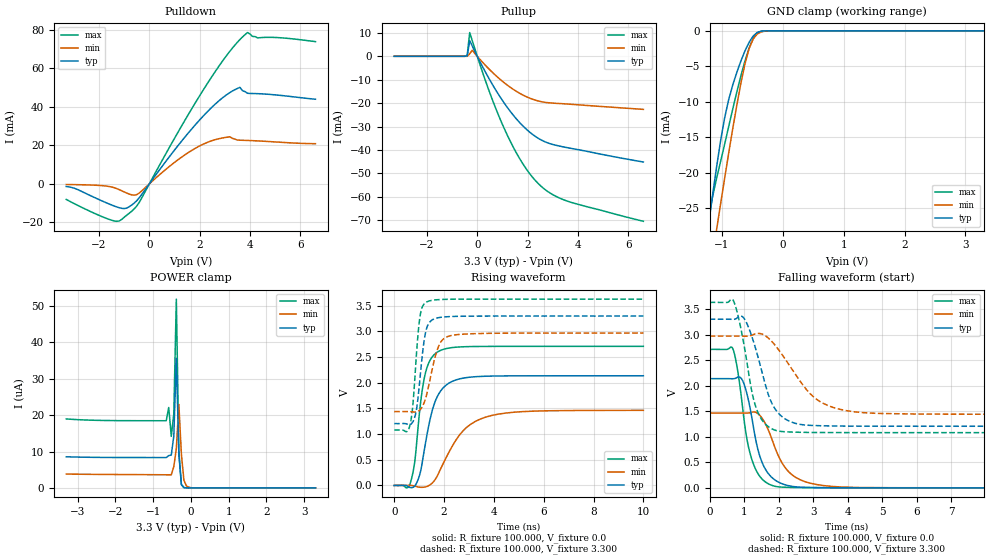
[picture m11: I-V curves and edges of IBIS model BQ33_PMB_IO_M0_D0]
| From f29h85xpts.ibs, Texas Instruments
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|   Model BQ33_PMB_IO_M0_D0
[Model]   BQ33_PMB_IO_M0_D0
Model_type   I/O
Polarity   Non-Inverting
Enable   Active-Low
Vinl =   0.990V
Vinh =   2.310V
Vmeas =  1.650V
Cref =   10.000pF
Vref =   0.0V
|   typ   min   max
C_comp   1.786pF   1.720pF   1.856pF
[Model Spec]
Vinh   2.310V   2.079V   2.541V
Vinl   0.990V   0.891V   1.089V
[Temperature Range]   30   155   -40
[Voltage Range]   3.300V   2.970V   3.630V
[Pullup Reference]   3.300V   2.970V   3.630V
[Pulldown Reference]   0.0V   0.0V   0.0V
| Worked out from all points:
|   slope of the pulldown table from 0 to 0.495 V, typ, clamps not added: 55.8 ohm
|   slope of the pullup table from 0 to 0.495 V, typ, clamps not added: 49.3 ohm
|   GND clamp passes 1 mA (typ) near -0.51 V on its own axis
|   rising waveform, R_fixture 100.000, V_fixture 0.0: 20-80 % time 590ps typ, 1.18ns min, 399ps max; typ from 0 V to 2.14 V
|   rising waveform, R_fixture 100.000, V_fixture 3.300: 20-80 % time 286ps typ, 457ps min, 238ps max; typ from 1.21 V to 3.3 V
|   falling waveform, R_fixture 100.000, V_fixture 0.0: 20-80 % time 441ps typ, 650ps min, 388ps max; typ from 2.14 V to 0 V
|   falling waveform, R_fixture 100.000, V_fixture 3.300: 20-80 % time 565ps typ, 1.03ns min, 431ps max; typ from 3.3 V to 1.21 V
[Pulldown]
|Voltage   I(typ)   I(min)   I(max)
-3.3V     -1.377mA   -342.6uA   -8.105mA
-1.6V     -10.44mA   -1.363mA   -18.44mA
-1.1V     -12.71mA   -3.581mA   -18.49mA
-500mV    -8.748mA   -5.592mA   -11.5mA
1.3V      22.5mA     14.05mA    30.49mA
2.5V      39.99mA    22.49mA    56.04mA
3.2V      47.44mA    24.45mA    68.91mA
3.5V      49.58mA    22.74mA    73.6mA
3.8V      47.94mA    22.6mA     77.52mA
3.9V      47.06mA    22.56mA    78.61mA
4.3V      46.87mA    22.32mA    75.86mA
6.6V      43.98mA    20.88mA    73.9mA
[Pullup]
|Voltage   I(typ)   I(min)   I(max)
-3.3V     194.8pA    13.15nA    1.362nA
-500mV    17.31nA    18.01nA    59.06nA
-400mV    178uA      374.8nA    408.1uA
-300mV    6.695mA    1.073mA    10.14mA
-200mV    4.421mA    2.585mA    6.742mA
400mV     -8.225mA   -4.706mA   -12.71mA
1V        -18.86mA   -10.69mA   -29.11mA
1.7V      -28.49mA   -15.89mA   -44mA
2.3V      -34.18mA   -18.71mA   -52.97mA
2.8V      -37mA      -19.82mA   -57.77mA
3.5V      -38.88mA   -20.34mA   -61.58mA
6.6V      -45.18mA   -22.68mA   -70.51mA
[GND_clamp]
|Voltage   I(typ)   I(min)   I(max)
-3.3V     -172.4mA   -157.9mA   -199.3mA
-1.223V   -27.66mA   -35.7mA    -26.88mA
-1.156V   -23.42mA   -31.92mA   -23.54mA
-1.089V   -19.35mA   -28.18mA   -20.9mA
-1.022V   -15.58mA   -24.48mA   -18.47mA
-955mV    -12.3mA    -20.84mA   -16.02mA
-821mV    -7.634mA   -13.8mA    -11.02mA
-620mV    -2.823mA   -4.656mA   -4.248mA
-553mV    -1.627mA   -2.518mA   -2.447mA
-419mV    -233.9uA   -454.3uA   -289uA
-218mV    -985nA     -9.253uA   -449.5nA
3.3V      0A         0A         0A
[POWER_clamp]
|Voltage   I(typ)   I(min)   I(max)
-3.3V     8.55uA     3.797uA    18.96uA
-653mV    8.339uA    3.596uA    18.47uA
-586mV    8.872uA    3.591uA    22.11uA
-519mV    9.031uA    3.588uA    14.17uA
-452mV    14.26uA    5.833uA    20.33uA
-385mV    35.62uA    10.82uA    51.91uA
-318mV    9.151uA    22.94uA    10.03uA
-251mV    942nA      9.217uA    856.3nA
-184mV    84.85nA    2.059uA    62.73nA
-117mV    8.015nA    524.6nA    4.599nA
-50mV     1.476nA    168.6nA    663.5pA
3.3V      0A         0A         0A
[Ramp]
| variable   typ   min   max
dV/dt_r   1.282/0.589n   0.878/1.174n   1.626/0.399n
dV/dt_f   1.257/0.565n   0.918/1.034n   1.530/0.430n
R_load = 100.000
[Rising Waveform]
R_fixture= 100.000
V_fixture= 0.0
V_fixture_min= 0.0
V_fixture_max= 0.0
|time   V(typ)   V(min)   V(max)
0s        15.47uV    20.08uV    14.59uV
641ps     -40.63mV   1.691mV    38.91mV
820ps     -12.29mV   -11.49mV   448.2mV
965ps     122.6mV    -30.55mV   1.173V
1.226ns   740.6mV    -31.31mV   2.133V
1.503ns   1.415V     36.93mV    2.49V
1.787ns   1.784V     243mV      2.614V
2.667ns   2.081V     1.01V      2.699V
3.652ns   2.128V     1.328V     2.709V
10ns      2.137V     1.464V     2.71V
[Rising Waveform]
R_fixture= 100.000
V_fixture= 3.300
V_fixture_min= 2.970
V_fixture_max= 3.630
|time   V(typ)   V(min)   V(max)
0s        1.205V     1.439V     1.08V
631ps     1.185V     1.438V     1.173V
745ps     1.237V     1.432V     1.545V
859ps     1.395V     1.43V      2.311V
1.028ns   2.051V     1.47V      3.263V
1.17ns    2.711V     1.576V     3.515V
1.308ns   3.071V     1.783V     3.575V
1.751ns   3.266V     2.673V     3.619V
2.181ns   3.289V     2.907V     3.627V
10ns      3.3V       2.97V      3.63V
[Falling Waveform]
R_fixture= 100.000
V_fixture= 0.0
V_fixture_min= 0.0
V_fixture_max= 0.0
|time   V(typ)   V(min)   V(max)
0s        2.137V     1.465V     2.71V
681ps     2.136V     1.465V     2.706V
935ps     2.122V     1.464V     1.682V
1.06ns    1.891V     1.464V     1.031V
1.185ns   1.514V     1.473V     639.7mV
1.44ns    649.3mV    1.428V     237.6mV
1.785ns   214mV      986.3mV    53.45mV
2.289ns   42.05mV    315.6mV    9.82mV
3.089ns   6.276mV    66.11mV    2.051mV
10ns      13.29uV    52.52uV    27.98uV
[Falling Waveform]
R_fixture= 100.000
V_fixture= 3.300
V_fixture_min= 2.970
V_fixture_max= 3.630
|time   V(typ)   V(min)   V(max)
0s        3.3V       2.97V      3.63V
695ps     3.298V     2.97V      3.653V
986ps     3.326V     2.969V     2.831V
1.331ns   2.726V     3.015V     1.597V
1.55ns    2.18V      3V         1.297V
1.861ns   1.581V     2.819V     1.138V
2.251ns   1.324V     2.457V     1.096V
2.9ns     1.224V     1.85V      1.085V
3.77ns    1.209V     1.537V     1.082V
10ns      1.205V     1.44V      1.08V
